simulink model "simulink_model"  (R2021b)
settings: Solver=VariableStepAuto  StartTime=0.0  StopTime=5  RelTol=1e-3

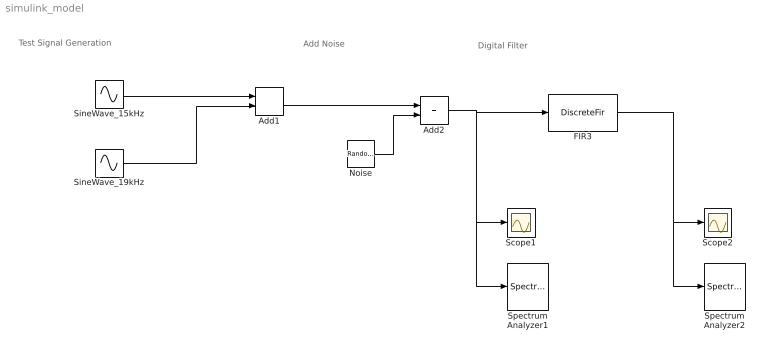
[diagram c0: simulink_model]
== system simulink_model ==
  note: Digital Filter
  note: Add Noise
  note: Test Signal Generation
  Add1 : Sum
  Add2 : Sum
  FIR3 : DiscreteFir  Tag=BlockMethodSubSystem  Coefficients=[0.00498579270301002103 0.00667954122285194934 0.00281316014875802357 -0.00772474614270733315 -0.0177129249699333989 -0.0170462175587224075 -0.00348252730831803085 0.0118064740257008208 0.0126963024641396152 -0.00470680358029653637 -0.0239142267917227397 -0.0215064853177068527 0.00710840552916844164 0.0361532540300490424 0.0299424660651754146 -0.0183480880844223218 -0.0672686013822251377 -0.053239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  InputProcessing=Columns as channels (frame based)
  Noise : RandomNumber  Variance=0.01  SampleTime=1/96e3
  Scope1 : Scope
  Scope2 : Scope
  SineWave_15kHz : Sin  Frequency=2*pi*15e3  SampleTime=1/96e3
  SineWave_19kHz : Sin  Frequency=2*pi*19e3  SampleTime=1/96e3
  Spectrum Analyzer1 : SpectrumAnalyzer
  Spectrum Analyzer2 : SpectrumAnalyzer
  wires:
  SineWave_15kHz/1 -> Add1/1
  SineWave_19kHz/1 -> Add1/2
  Add1/1 -> Add2/1
  Noise/1 -> Add2/2
  Add2/1 -> Scope1/1, Spectrum Analyzer1/1, FIR3/1
  FIR3/1 -> Scope2/1, Spectrum Analyzer2/1
